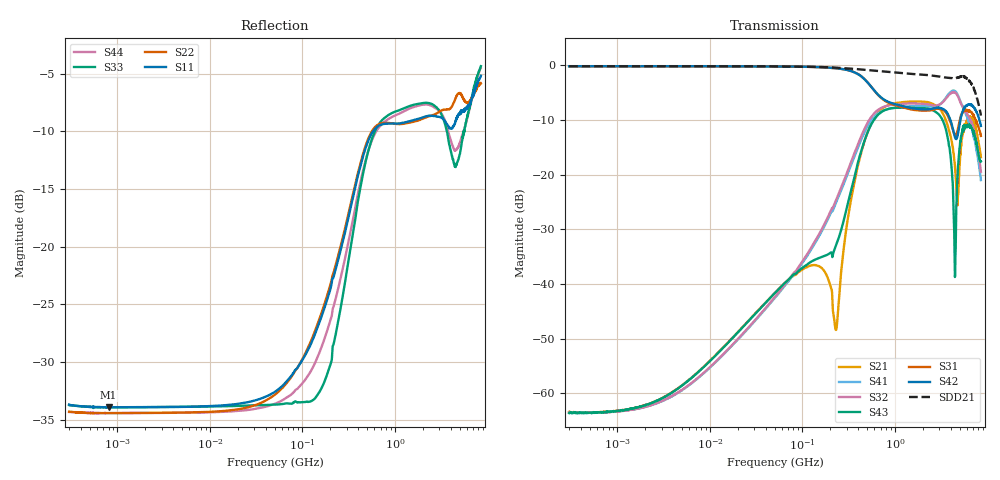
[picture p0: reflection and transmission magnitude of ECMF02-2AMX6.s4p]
!ECMF02-2AMX6
!Typical device
!10/03/10  11:16
!E5071BSP.exe
!Probes on PCB
!P1 Probe Type :ACP GSS-400; Probe S/N : 97237
!P2 Probe Type :ACP GSS-400; Probe S/N : 97237
!P3 Probe Type :ACP SSG-400; Probe S/N : 97238
!P4 Probe Type :ACP SSG-400; Probe S/N : 97238
! Instrument Manufacturer: Agilent Technologies
! Instrument Model: E5071B
! Instrument Serial Number: MY42301810
! Instrument Firmware Rev: A.08.11
!Start Freq. :300.000kHz; Stop Freq. : 8.500GHz
!Number of points : 1601; Sweep : LINEAR
!Ports power : 0.000000dBm; IFBW : 100.000000Hz
!Calibration kit : 106-683 (22832)
!Prober : PM8 (Manual prober)
!Darkness measurement :NO
!Voltage measurement :NO
!Temperature measurement :NO
!Lane 1 or 2
! Freq ReS11 ImS11 ReS12 ImS12 ReS13 ImS13 ReS14 ImS14
!  ReS21 ImS21 ReS22 ImS22 ReS23 ImS23 ReS24 ImS24
!  ReS31 ImS31 ReS32 ImS32 ReS33 ImS33 ReS34 ImS34
!  ReS41 ImS41 ReS42 ImS42 ReS43 ImS43 ReS44 ImS44
# Hz  S  RI  R  50
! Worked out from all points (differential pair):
!   1601 points, 300 kHz to 8.5 GHz, reference 50 ohm
!   strongest paths, dB at 300 kHz, 3.892 MHz, 50.5 MHz, 655.2 MHz, 8.5 GHz:
!     S42: -0.2, -0.2, -0.2, -5.3, -11.1
!     S31: -0.2, -0.2, -0.2, -5.4, -12.9
!     S43: -63.6, -59.8, -41.6, -9.1, -17.6
!     S32: -63.4, -60.5, -42.4, -8.2, -19.5
!     S41: -63.6, -60.5, -42.5, -8.8, -21.0
!     S21: -63.4, -59.8, -41.6, -8.7, -16.8
!   taken as a pair (ports 2,1 in; 4,3 out), SDD21 dB: -0.2, -0.2, -0.2, -1.0, -9.2
!   lowest |S11| = -33.9 dB at 802.1 kHz (marker M1), VSWR 1.04, Z = 52.1 - j0.022 ohm
!   |S11| at or under -10 dB: start of sweep to 581.2 MHz
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300000  0.0207 -0.000184  0.000672 8.71e-05  0.9804 -0.00105  -0.000667 -8.01e-05
        0.000673 8.7e-05  0.0193 -0.000127  -0.000668 -7.27e-05  0.9809 -0.000567
        0.9799 -0.000771  -0.000668 -8.01e-05  0.0206 -0.000162  0.000661 8.48e-05
        -0.000659 -8.35e-05  0.9802 -0.00174  0.000656 8.91e-05  0.0192 -0.000196
802088.4  0.0201 -0.000211  0.000657 0.000167  0.9804 -0.0026  -0.000657 -0.000149
          0.000661 0.000171  0.019 -0.000122  -0.000659 -0.000145  0.9805 -0.00212
          0.9786 -0.00224  -0.000659 -0.000143  0.0202 -0.000128  0.000653 0.000177
          -0.000664 -0.000147  0.9817 -0.00268  0.000659 0.000169  0.019 -0.000133
2.299082e8  0.00854 -0.08  0.00251 -0.00281  0.7295 -0.5954  -0.037 -0.0411
            0.00248 -0.00288  -0.0177 -0.0819  -0.05 -0.03  0.7267 -0.5967
            0.7282 -0.5949  -0.0498 -0.0298  -0.0241 -0.0345  -0.0121 0.0191
            -0.0369 -0.0409  0.7268 -0.5982  -0.012 0.0188  -0.027 -0.0536
6.59367e8  -0.2443 0.2266  -0.0811 0.3615  -0.0997 -0.5272  -0.1396 0.3332
           -0.0806 0.3621  -0.176 0.2889  -0.0656 0.3885  -0.098 -0.5291
           -0.098 -0.5255  -0.0673 0.3864  -0.0386 0.3342  0.0397 0.3494
           -0.1394 0.3356  -0.0966 -0.5291  0.0408 0.352  -0.1098 0.3065
3.813715e9  0.0028 -0.331  0.1609 -0.2036  0.0563 0.3255  0.3994 -0.3727
            0.1634 -0.2012  -0.0274 -0.3927  0.3753 -0.3914  0.0934 0.3267
            0.0599 0.3252  0.3703 -0.3843  -0.0236 -0.2851  0.1006 -0.1678
            0.4009 -0.3747  0.1027 0.3296  0.099 -0.1658  -0.00567 -0.3097
4.429426e9  -0.2295 -0.2532  0.00865 -0.1253  0.0637 0.2297  0.1737 -0.5504
            0.0107 -0.1269  -0.2607 -0.3421  0.1551 -0.5575  0.1067 0.2076
            0.0694 0.2219  0.1599 -0.5447  -0.2035 -0.0911  -0.00738 -0.0215
            0.1641 -0.5567  0.1087 0.1949  -0.00408 -0.0145  -0.2113 -0.1538
8.5e9  0.413 0.3632  0.1366 0.0225  0.2057 -0.1046  -0.086 0.0321
       0.1437 0.0172  0.3988 0.318  -0.0986 0.0578  0.2056 -0.1867
       0.2078 -0.0891  -0.0956 0.0468  0.5663 0.214  0.0976 0.0684
       -0.0807 0.0381  0.2128 -0.1806  0.1123 0.0694  0.5935 0.0581
